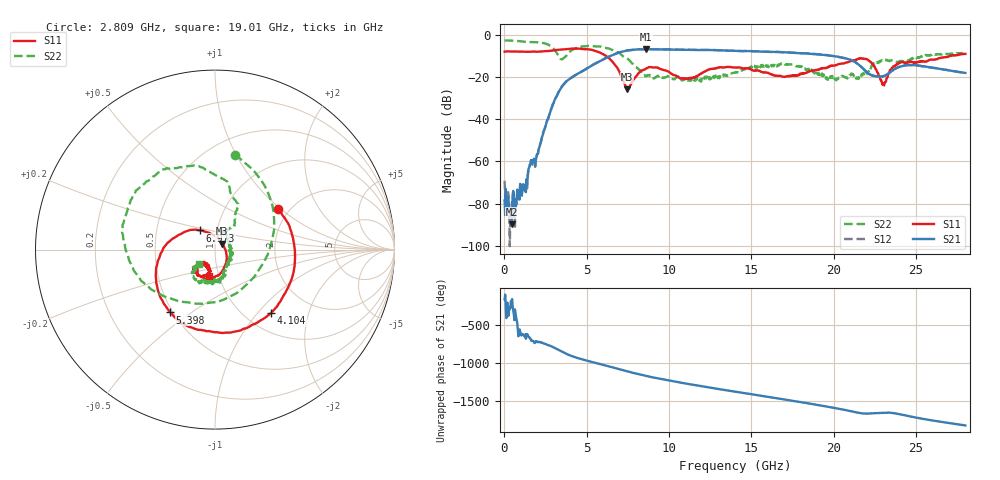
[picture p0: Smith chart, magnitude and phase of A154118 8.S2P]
!  2-Port S-parameters saved by WinCal
! VAR MeasName=S-Parameters (CALIBRATED_DATA) read from VNA (N5230A)
! VAR MeasDate=2015-9-10 14:35:00
! VAR NAME=A154118 8
! VAR FILENAME=A154118 8.S2P
! VAR DATE=2015-9-10 14:35:00
! VAR PHYS_PORTS=1,2
# Hz S DB R 50
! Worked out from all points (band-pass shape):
!   801 points, 10 MHz to 28 GHz, reference 50 ohm
!   highest |S21| = -6.81 dB at 8.582 GHz (marker M1); lowest = -89.8 dB at 429.9 MHz (marker M2)
!   |S21| within 3 dB of the highest: 6.502 GHz to 19.71 GHz (13.2 GHz wide, 101 % of centre)
!   lowest |S11| = -25.8 dB at 7.462 GHz (marker M3), VSWR 1.11, Z = 54 + j3.55 ohm
!   |S11| at or under -10 dB: 6.16 GHz to 27.05 GHz (20.89 GHz wide, 126 % of centre)
!   |S22| runs from -22.2 to -2.7 dB; largest |S21 - S12| = 0.0086
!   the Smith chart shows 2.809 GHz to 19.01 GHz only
!   S11 on the Smith chart (normalised r, x): 2.809 GHz: 1.75, +0.96; 4.104 GHz: 1.30, -1.18; 5.398 GHz: 0.48, -0.42; 6.973 GHz: 0.83, +0.18; 19.01 GHz: 0.90, -0.27
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1e7  -7.97 179.5  -78.51 -154.6  -69.21 -129.8  -2.66 179.8
4.2985e8  -7.89 159.4  -89.80 153.9  -83.21 36.5  -2.75 169.5
1.26955e9  -8.02 119.5  -74.22 100.4  -74.20 82.8  -3.33 149.2
2.809e9  -7.57 32.7  -35.84 -52.4  -35.85 -52.0  -5.38 78.2
3.298825e9  -7.07 1.7  -27.03 -104.6  -26.99 -104.5  -10.18 3.8
3.6487e9  -6.79 -20.5  -22.96 -143.8  -22.94 -143.6  -10.69 -88.0
4.103538e9  -6.53 -48.6  -20.12 173.6  -20.11 173.9  -7.17 -154.9
4.698325e9  -6.62 -84.9  -17.43 131.8  -17.39 131.9  -5.52 166.3
5.398075e9  -7.34 -125.5  -14.14 91.4  -14.07 91.5  -5.39 136.4
6.972512e9  -17.36 127.9  -8.39 0.8  -8.32 0.4  -8.62 77.8
7.462338e9  -25.83 39.9  -7.41 -28.4  -7.38 -28.6  -11.29 61.3
8.581938e9  -16.11 -93.7  -6.81 -87.6  -6.77 -87.9  -19.65 56.8
9.351662e9  -15.71 -126.1  -6.93 -122.5  -6.85 -122.8  -19.48 68.7
1.1206e10  -20.61 -119.5  -7.13 164.1  -7.08 163.4  -21.33 21.2
1.4005e10  -15.50 -128.7  -7.59 64.2  -7.57 63.6  -17.95 -63.7
1.627919e10  -18.82 -134.9  -8.13 -13.4  -8.14 -14.1  -14.34 -107.1
1.869332e10  -16.91 -101.2  -9.02 -99.8  -9.03 -100.2  -16.73 -134.6
1.900821e10  -16.46 -101.9  -9.23 -111.7  -9.20 -112.1  -18.45 -137.2
2.170225e10  -11.27 -122.9  -15.37 137.9  -15.29 136.8  -18.63 -89.8
2.299679e10  -23.07 -118.4  -19.66 144.6  -19.71 144.0  -11.96 -88.8
2.334666e10  -18.19 -82.0  -18.25 146.3  -18.21 145.9  -12.33 -94.7
2.8e10  -9.04 -111.4  -18.07 -22.9  -18.09 -23.4  -8.43 -121.0
